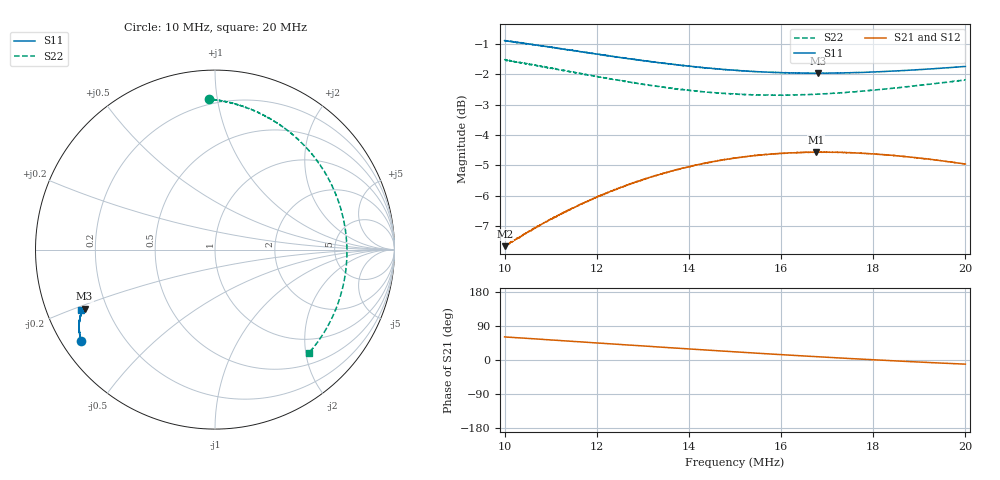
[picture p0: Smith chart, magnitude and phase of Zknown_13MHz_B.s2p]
!Agilent Technologies,N5242A,MY49421279,A.09.90.21
!Agilent N5242A: A.09.90.21
!Date: Monday, January 30, 2023
!Caliblation kit: 85033D 3.5mm Calibration Kit
!DUT Connector Gender Port1: male
!DUT Connector Gender Port2: female
!S2P File: Measurements: S11, S21, S12, S22:
# Hz S  dB  R 50
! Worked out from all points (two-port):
!   2001 points, 10 MHz to 20 MHz, reference 50 ohm
!   highest |S21| = -4.56 dB at 16.76 MHz (marker M1); lowest = -7.7 dB at 10.01 MHz (marker M2)
!   |S21| within 3 dB of the highest: 10.12 MHz to end of sweep
!   lowest |S11| = -2.0 dB at 16.8 MHz (marker M3), VSWR 8.88, Z = 5.89 - j10.6 ohm
!   |S11| at or under -10 dB: nowhere
!   |S22| runs from -2.7 to -1.5 dB; largest |S21 - S12| = 0.0024
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1e7  -0.89 -145.6  -7.65 61.0  -7.69 60.9  -1.53 92.5
1.0005e7  -0.89 -145.7  -7.66 60.9  -7.68 60.9  -1.51 92.4
1.038e7  -0.96 -147.1  -7.32 57.9  -7.34 57.9  -1.61 87.7
1.0825e7  -1.07 -148.6  -6.93 54.4  -6.94 54.4  -1.75 81.8
1.126e7  -1.16 -149.9  -6.56 51.0  -6.58 51.0  -1.86 75.9
1.167e7  -1.25 -151.0  -6.27 47.7  -6.28 47.8  -1.98 70.2
1.215e7  -1.36 -152.2  -5.95 43.8  -5.95 43.9  -2.10 63.3
1.253e7  -1.45 -152.8  -5.72 40.8  -5.73 40.9  -2.20 57.7
1.3335e7  -1.60 -154.1  -5.32 34.4  -5.30 34.5  -2.39 45.5
1.4185e7  -1.75 -155.0  -4.98 27.8  -4.97 27.8  -2.55 32.3
1.463e7  -1.82 -155.2  -4.84 24.3  -4.84 24.4  -2.62 25.3
1.5e7  -1.86 -155.4  -4.76 21.5  -4.76 21.6  -2.65 19.5
1.538e7  -1.90 -155.5  -4.68 18.7  -4.67 18.8  -2.67 13.6
1.5825e7  -1.93 -155.6  -4.62 15.4  -4.61 15.5  -2.68 6.8
1.6225e7  -1.95 -155.7  -4.59 12.5  -4.58 12.6  -2.68 0.7
1.667e7  -1.96 -155.6  -4.56 9.5  -4.55 9.4  -2.66 -5.8
1.676e7  -1.96 -155.6  -4.56 8.9  -4.55 8.8  -2.65 -7.1
1.6795e7  -1.96 -155.6  -4.56 8.6  -4.56 8.6  -2.64 -7.6
1.7505e7  -1.94 -155.6  -4.59 3.8  -4.58 3.8  -2.58 -17.5
1.8335e7  -1.89 -155.6  -4.65 -1.4  -4.65 -1.4  -2.47 -28.4
1.921e7  -1.82 -155.7  -4.79 -6.6  -4.79 -6.7  -2.32 -39.0
2e7  -1.74 -155.8  -4.95 -10.9  -4.96 -11.0  -2.18 -47.7
